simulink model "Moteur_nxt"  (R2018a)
settings: Solver=FixedStepAuto  StartTime=0.0  StopTime=inf  RelTol=1e-3  EnableMultiTasking=on
libraries: arduinolib x2, simulink x1

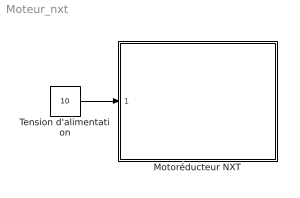
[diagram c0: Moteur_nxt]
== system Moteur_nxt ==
  Motoréducteur NXT : Subsystem
  Tension d'alimentation : Constant  Value=10
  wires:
  Tension d'alimentation/1 -> Motoréducteur NXT/1(U)

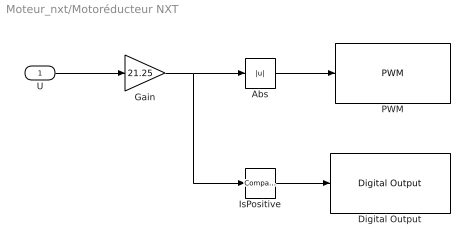
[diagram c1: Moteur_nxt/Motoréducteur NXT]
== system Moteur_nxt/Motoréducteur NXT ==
  U : Inport
  Abs : Abs
  Digital Output : arduinolib/Digital Output  pinNumber=12  blockPlatform=arduino
  Gain : Gain  Gain=21.25
  IsPositive : simulink/Logic and Bit Operations/Compare To Zero  relop=>  OutDataTypeStr=boolean
  PWM : arduinolib/PWM  pinNumber=3  EnableInputFrequency=off  InitialFrequency=2000  InitialDutyCycle=0  NotificationType=None  blockPlatform=arduino
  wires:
  IsPositive/1 -> Digital Output/1
  U/1 -> Gain/1
  Gain/1 -> IsPositive/1, Abs/1
  Abs/1 -> PWM/1
